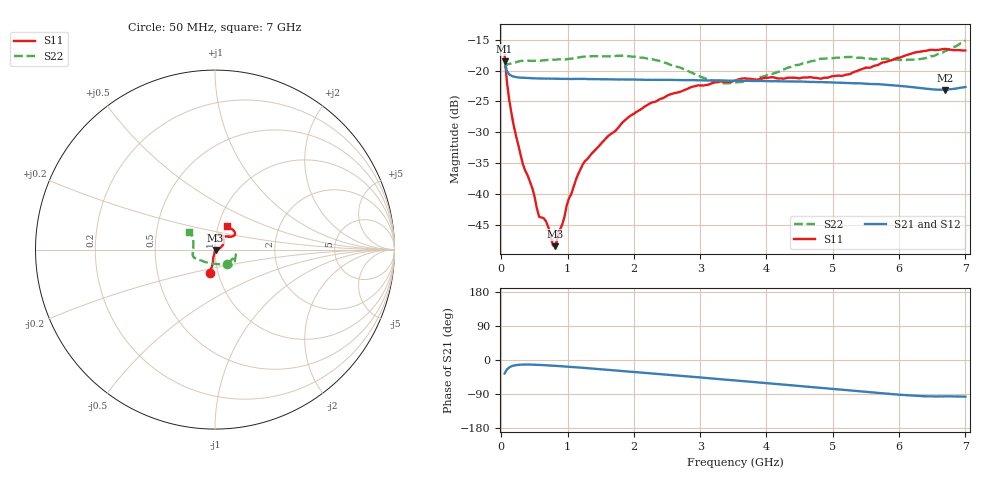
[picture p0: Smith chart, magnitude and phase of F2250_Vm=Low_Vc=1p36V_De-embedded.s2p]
! Integrated Device Technology
! Corporate Headquarters
! 6024 Silver Creek Valley Road
! San Jose, CA 95138  USA
! Phone:  1-408-284-8200
! Toll Free:  1-800-223-1366
! Webpage:  http://www.idt.com/
! Timing and RF Division
! 515 Groton Road, Suite 102
! Westford, MA 01886-6024
! Device:  F2250
! Description: Voltage Variable RF Attenuator
! Frequency:  50.0 -  6000.00 MHz
! Package:  3x3 mm Thin QFN Plastic Package: 16 pin
! Ports:  2 RF, 3 DC
!  Pin  1  = GND
!  Pin  2  = NC
!  Pin  3  = RF1  = Port 1
!  Pin  4  = NC
!  Pin  5  = GND
!  Pin  6  = GND
!  Pin  7  = GND
!  Pin  8  = GND
!  Pin  9  = NC
!  Pin 10  = RF2  = Port 2
!  Pin 11  = NC
!  Pin 12  = GND
!  Pin 13  = GND
!  Pin 14  = VCNTRL
!  Pin 15  = VDD
!  Pin 16  = VMODE
! Vcntrl:  1.360 Volts
! Vmode:  +0.000 Volts
! Vdd:  +3.30  Volts
! Current:  1.193 mA
! Data:  The device was measured on a the F2250 evaluation board which has
!  individual transmission lines to the RF pins.  Data was collected
!  using a calibrated network analyzer.  The evaluation board was
!  de-embedded using a TRL calibration technique.
!  The reference plane is the edge of the package pin.
! Misc:  SN 10
!  Action Tracker AT0258
! Date Measured:  2014-11-26
! Date:  2015-10-15  MJV
! Note:
!  Integrated Device Technology supplies this data as a sample of measured
!  data at the package pin for this product.  Your particular data for this
!  product may vary.
!  Data was taken at 25 degrees C.
!  Integrated Device Technology reserves the right to change this data at anytime.
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# GHz S dB R 50
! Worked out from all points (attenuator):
!   201 points, 50 MHz to 7 GHz, reference 50 ohm
!   highest |S21| = -18.50 dB at 50 MHz (marker M1); lowest = -23.1 dB at 6.687 GHz (marker M2)
!   lowest |S11| = -48.5 dB at 814.5 MHz (marker M3), VSWR 1.01, Z = 50.3 - j0.214 ohm
!   |S11| at or under -10 dB: start of sweep to end of sweep
!   |S22| runs from -22.1 to -15.1 dB; largest |S21 - S12| = 0.00035
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0.05  -17.52 -103.0  -18.50 -35.5  -18.52 -35.6  -19.56 -49.5
0.08475  -21.85 -98.8  -20.08 -25.1  -20.10 -25.1  -19.00 -25.6
0.15425  -27.03 -101.9  -20.85 -16.5  -20.87 -16.5  -18.85 -15.4
0.328  -35.28 -99.4  -21.18 -12.0  -21.17 -12.0  -18.43 -13.3
0.467  -39.06 -100.8  -21.25 -12.2  -21.25 -12.2  -18.44 -14.7
0.57125  -43.74 -88.5  -21.29 -12.9  -21.29 -12.9  -18.41 -17.2
0.6755  -44.48 -72.8  -21.31 -13.9  -21.30 -13.9  -18.30 -19.4
0.77975  -48.39 -45.8  -21.33 -15.0  -21.32 -15.0  -18.27 -21.9
0.8145  -48.50 -34.5  -21.33 -15.4  -21.32 -15.4  -18.24 -22.9
1.023  -40.69 -14.5  -21.37 -17.9  -21.37 -17.9  -18.11 -26.9
1.2315  -35.17 4.0  -21.36 -20.6  -21.37 -20.6  -17.77 -31.3
1.9265  -27.49 25.5  -21.46 -30.4  -21.45 -30.4  -17.69 -40.5
2.37825  -24.73 35.6  -21.53 -36.8  -21.53 -36.8  -18.40 -47.2
2.86475  -22.69 49.3  -21.56 -44.1  -21.57 -44.1  -20.32 -61.0
3.14275  -22.23 56.6  -21.60 -48.2  -21.58 -48.2  -21.52 -75.7
3.525  -21.62 66.9  -21.66 -53.9  -21.68 -53.9  -21.94 -102.8
4.7065  -21.17 69.6  -21.85 -72.0  -21.85 -72.0  -18.44 -156.0
5.15825  -20.82 54.6  -22.00 -79.0  -22.01 -79.0  -17.84 -164.0
5.85325  -18.42 37.5  -22.36 -89.5  -22.37 -89.5  -18.15 -176.7
6.305  -16.97 38.5  -22.82 -95.1  -22.83 -95.1  -18.16 166.9
6.68725  -16.50 47.3  -23.14 -95.9  -23.14 -95.9  -16.87 150.0
7  -16.75 62.7  -22.66 -96.7  -22.65 -96.8  -15.12 145.9
